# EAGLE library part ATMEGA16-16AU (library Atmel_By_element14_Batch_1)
8-bit Microcontroller
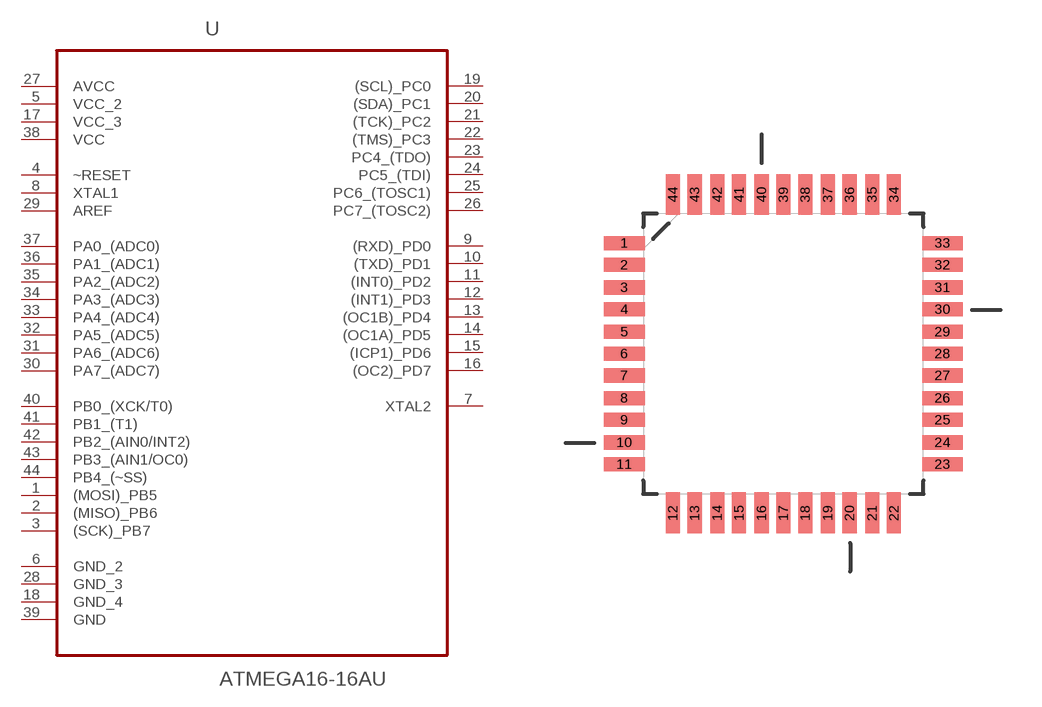
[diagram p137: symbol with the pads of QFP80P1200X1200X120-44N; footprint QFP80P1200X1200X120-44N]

Designator prefix U

## ATMEGA16-16AU (DESCRIPTION: 8-bit Microcontroller; MPN: ATMEGA16-16AU; OC_FARNELL: 9171134; OC_NEWARK: 96K6515; PACKAGE: QFP-44; SUPPLIER: Atmel)  [QFP80P1200X1200X120-44N]
1  (MOSI)_PB5
2  (MISO)_PB6
3  (SCK)_PB7
4  ~RESET  in
5  VCC_2  pwr
6  GND_2  pas
7  XTAL2  out
8  XTAL1  in
9  (RXD)_PD0
10  (TXD)_PD1
11  (INT0)_PD2
12  (INT1)_PD3
13  (OC1B)_PD4
14  (OC1A)_PD5
15  (ICP1)_PD6
16  (OC2)_PD7
17  VCC_3  pwr
18  GND_4  pas
19  (SCL)_PC0
20  (SDA)_PC1
21  (TCK)_PC2
22  (TMS)_PC3
23  PC4_(TDO)
24  PC5_(TDI)
25  PC6_(TOSC1)
26  PC7_(TOSC2)
27  AVCC  pwr
28  GND_3  pas
29  AREF  in
30  PA7_(ADC7)
31  PA6_(ADC6)
32  PA5_(ADC5)
33  PA4_(ADC4)
34  PA3_(ADC3)
35  PA2_(ADC2)
36  PA1_(ADC1)
37  PA0_(ADC0)
38  VCC  pwr
39  GND  pas
40  PB0_(XCK/T0)
41  PB1_(T1)
42  PB2_(AIN0/INT2)
43  PB3_(AIN1/OC0)
44  PB4_(~SS)

## Footprint QFP80P1200X1200X120-44N (pad centres in mm)
smd 1.473 x 0.508: 1 -5.74,3.988; 2 -5.74,3.2; 3 -5.74,2.388; 4 -5.74,1.6; 5 -5.74,0.787; 6 -5.74,0; 7 -5.74,-0.787; 8 -5.74,-1.6; 9 -5.74,-2.388; 10 -5.74,-3.2; 11 -5.74,-3.988; 23 5.74,-3.988; 24 5.74,-3.2; 25 5.74,-2.388; 26 5.74,-1.6; 27 5.74,-0.787; 28 5.74,0; 29 5.74,0.787; 30 5.74,1.6; 31 5.74,2.388; 32 5.74,3.2; 33 5.74,3.988
smd 0.508 x 1.473: 12 -3.988,-5.74; 13 -3.2,-5.74; 14 -2.388,-5.74; 15 -1.6,-5.74; 16 -0.787,-5.74; 17 0,-5.74; 18 0.787,-5.74; 19 1.6,-5.74; 20 2.388,-5.74; 21 3.2,-5.74; 22 3.988,-5.74; 34 3.988,5.74; 35 3.2,5.74; 36 2.388,5.74; 37 1.6,5.74; 38 0.787,5.74; 39 0,5.74; 40 -0.787,5.74; 41 -1.6,5.74; 42 -2.388,5.74; 43 -3.2,5.74; 44 -3.988,5.74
